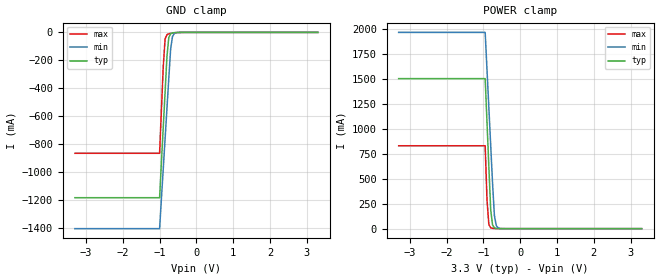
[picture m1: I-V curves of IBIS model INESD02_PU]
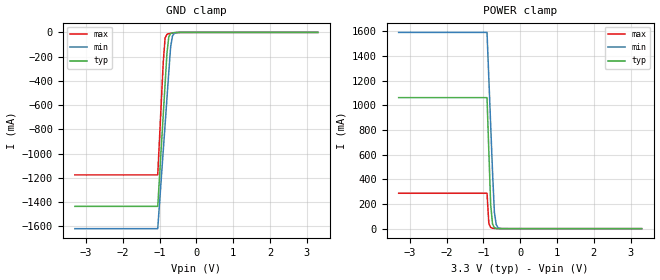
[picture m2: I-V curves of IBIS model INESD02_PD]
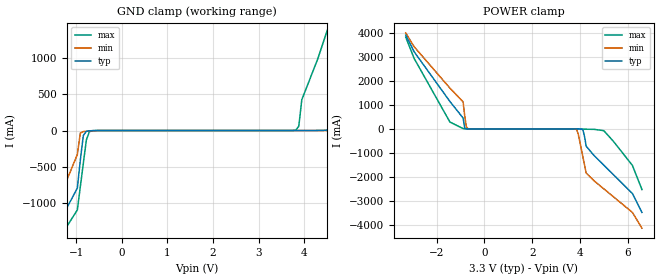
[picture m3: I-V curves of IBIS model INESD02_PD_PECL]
|   This file is an IBIS representation of the   |
|   Integrated Device Technology, Inc.   |
|   ICS85105I   |
|   Low Skew, 1-to-5, Differential/LVCMOS-to-0.7V HCSL Fanout Buffer   |
[IBIS Ver]   4.1
[File name]   85105i_3v3.ibs
[File Rev]   4.0
[Date]   27 Aug 2009 | Last modified
|   May 07 2007 | Generated
[Source]   Originated at Integrated Device Technology, Inc.
[Disclaimer]
IDT hereby grants the user of this IBIS model a non-exclusive,
nontransferable license to use this IBIS model under the following terms.
Before using this IBIS model, the user should read this license.
If the user does not accept these terms,  the IBIS model should be
returned to IDT within 30 days.
   The user is granted this license only to use the IBIS model and
is not granted rights to sell, load, rent, lease or license the IBIS
model in whole or in part, or in modified form to anyone other than
user. User may modify the IBIS model to suit its specific
applications but rights to derivative works and such modifications
shall belong to IDT.
   This IBIS model is provided on an "AS IS" basis and IDT makes
absolutely no warranty with respect to the information contained
herein. IDT DISCLAIMS AND CUSTOMER WAIVES ALL WARRANTIES, EXPRESS
OR IMPLIED, INCLUDING WARRANTIES OF MERCHANTABILITY OR FITNESS FOR
A PARTICULAR PURPOSE. The entire risk as to quality and performance
is with the Customer. ACCORDINGLY, IN NO EVENT SHALL THE COMPANY BE
LIABLE FOR ANY DAMAGES, WHETHER IN CONTRACT OR TORT,INCLUDING ANY
LOST PROFITS OR OTHER INCIDENTAL, CONSEQUENTIAL, EXEMPLARY, OR
PUNITIVE DAMAGES ARISING OUT OF THE USE OR APPLICATION OF THE IBIS
model provided in this package. Further, IDT reserves the right to
make changes without notice to any product herein to improve
reliability, function, or design. IDT does not convey any license
under patent rights or any other intellectual property rights,
including those of third parties.
   IDT is not obligated to provide maintenance or support
for the licensed IBIS model.
[Copyright]   Copyright 2006 by Integrated Device Technology, Inc.
[Component]   ICS85105GI
[Manufacturer] Integrated Device Technology, Inc.
[Package]
|TSSOP 20 Lead
|   typ   min   max
R_pkg   51.85m   41.1m   62.6m
L_pkg   1.568nH   0.734nH   2.401nH
C_pkg   0.221pF   0.068pF   0.373pF
[Pin] signal_name  model_name   R_pin   L_pin   C_pin
1   GND   GND   62.6m   2.401n   0.373p
2   CLK_EN   INESD02_PU   57.23m   1.985n   0.297p
3   CLK_SEL   INESD02_PD   51.85m   1.568n   0.221p
4   CLK0   INESD02_PD_PECL   46.78m   1.151n   0.145p
5   nCLK0   INESD02_PD_PU   41.1m   0.734n   0.068p
6   CLK1   INESD02_PD_PECL   41.1m   0.734n   0.068p
7   Q4   DCMOUT01_ISO2_OP   46.78m   1.151n   0.145p
8   nQ4   DCMOUT01_ISO2_OP   51.85m   1.568n   0.221p
9   IREF   NC   57.23m   1.985n   0.297p
10  VDD   POWER   62.6m   2.401n   0.373p
11  nQ3   DCMOUT01_ISO2_OP   62.6m   2.401n   0.373p
12  Q3   DCMOUT01_ISO2_OP   57.23m   1.985n   0.297p
13  VDD   POWER   51.85m   1.568n   0.221p
14  nQ2   DCMOUT01_ISO2_OP   46.78m   1.151n   0.145p
15  Q2   DCMOUT01_ISO2_OP   41.1m   0.734n   0.068p
16  nQ1   DCMOUT01_ISO2_OP   41.1m   0.734n   0.068p
17  Q1   DCMOUT01_ISO2_OP   46.78m   1.151n   0.145p
18  VDD   POWER   51.85m   1.568n   0.221p
19  nQ0   DCMOUT01_ISO2_OP   57.23m   1.985n   0.297p
20  Q0   DCMOUT01_ISO2_OP   62.6m   2.401n   0.373p
[Diff Pin]   inv_pin  vdiff tdelay_typ tdelay_min  tdelay_max
   4   5   0.15   0   0   0
   20   19   NA   0   0   0
   17   16   NA   0   0   0
   15   14   NA   0   0   0
   12   11   NA   0   0   0
   7   8   NA   0   0   0
| Models and submodels in the file (5): INESD02_PU (Input), INESD02_PD (Input), INESD02_PD_PECL (Input), INESD02_PD_PU (Input), DCMOUT01_ISO2_OP (Open_source)
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[Model]   INESD02_PU
Model_type   Input
Polarity   Non-Inverting
Vinl = 0.80V
Vinh = 2.0V
|   typ   min   max
C_comp   2pF   1.5pF   2.5pF
|   typ   min   max
[Voltage range]  3.3V   3.15V   3.45V
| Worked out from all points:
|   GND clamp passes 1 mA (typ) near -0.56 V on its own axis
|   POWER clamp passes 1 mA (typ) near -0.61 V on its own axis
[GND_clamp]
|Voltage   I(typ)   I(min)   I(max)
-3.3V     -1.184A    -1.405A    -865.6mA
-1V       -1.184A    -1.405A    -865.6mA
-900mV    -678.5mA   -975.1mA   -244.1mA
-850mV    -426.2mA   -760.2mA   -46.92mA
-800mV    -174mA     -545.4mA   -16.17mA
-750mV    -37.03mA   -330.8mA   -9.981mA
-700mV    -9.767mA   -120.3mA   -7.122mA
-650mV    -3.616mA   -29.78mA   -4.922mA
-600mV    -1.7mA     -7.594mA   -3.115mA
-400mV    -123.9uA   -126uA     -173.9uA
3.3V      1.866nA    3.949uA    0A
[POWER_clamp]
|Voltage   I(typ)   I(min)   I(max)
-3.3V     1.506A     1.97A      832.1mA
-950mV    1.506A     1.97A      832.1mA
-900mV    1.063A     1.592A     287.2mA
-850mV    620.4mA    1.215A     41.77mA
-800mV    191.5mA    837.4mA    8.692mA
-750mV    37.69mA    460.1mA    3.262mA
-700mV    8.032mA    133.8mA    1.662mA
-650mV    2.005mA    32.58mA    840.1uA
-600mV    607uA      8.009mA    378.6uA
-450mV    33.11uA    139.8uA    23.88uA
3.3V      -71.13uA   -77.46uA   -62.11uA
[Model]   INESD02_PD
Model_type   Input
Polarity   Non-Inverting
Vinl = 0.80V
Vinh = 2.0V
|   typ   min   max
C_comp   2pF   1.5pF   2.5pF
|   typ   min   max
[Voltage range]  3.3V   3.15V   3.45V
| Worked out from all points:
|   GND clamp passes 1 mA (typ) near -0.56 V on its own axis
|   POWER clamp passes 1 mA (typ) near -0.61 V on its own axis
[GND_clamp]
|Voltage   I(typ)   I(min)   I(max)
-3.3V     -1.436A    -1.62A     -1.176A
-1.05V    -1.436A    -1.62A     -1.176A
-900mV    -678.5mA   -975.1mA   -244mA
-850mV    -426.1mA   -760.1mA   -46.85mA
-800mV    -173.9mA   -545.4mA   -16.11mA
-750mV    -36.96mA   -330.7mA   -9.916mA
-700mV    -9.696mA   -120.2mA   -7.056mA
-650mV    -3.545mA   -29.7mA    -4.857mA
-600mV    -1.629mA   -7.52mA    -3.049mA
-400mV    -52.81uA   -52.52uA   -108.7uA
3.3V      71.13uA    77.43uA    62.11uA
[POWER_clamp]
|Voltage   I(typ)   I(min)   I(max)
-3.3V     1.063A     1.593A     287.3mA
-900mV    1.063A     1.593A     287.3mA
-850mV    620.5mA    1.215A     41.84mA
-800mV    191.6mA    837.5mA    8.757mA
-750mV    37.76mA    460.2mA    3.328mA
-700mV    8.104mA    133.8mA    1.728mA
-650mV    2.076mA    32.66mA    905.3uA
-600mV    678.1uA    8.083mA    443.8uA
-450mV    104.2uA    213.3uA    89.09uA
3.3V      -3.041nA   -3.986uA   0A
[Model]   INESD02_PD_PECL
Model_type  Input
Polarity   Non-Inverting
Vinl = 0.8V
Vinh = 2.0V
|   typ   min   max
C_comp   2pF   1.5pF   2.5pF
|   typ   min   max
[Voltage range]  3.3V   3.15V   3.45V
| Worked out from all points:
|   GND clamp passes 1 mA (typ) near -0.59 V on its own axis
|   POWER clamp passes 1 mA (typ) near -0.70 V on its own axis
[GND_clamp]
-3.3V     -3.894A    -4.294A    -3.674A
-1.6V     -1.569A    -1.322A    -1.74A
-974.8mV  -794.1mA   -331.5mA   -1.096A
-843.4mV  -68.33mA   -15.34mA   -452.9mA
-646.5mV  -1.912mA   -4.151mA   -2.665mA
3.818V    89.38uA    70.49uA    7.198mA
3.95V     342.2uA    75.94uA    423.8mA
4.6V      7.437mA    165.5uA    1.553A
4.9V      78.32mA    440.9uA    2.118A
5.5V      1.293A     2.769mA    3.249A
6.25V     2.651A     112.4mA    4.38A
6.6V      3.331A     896.1mA    4.946A
[POWER_clamp]
-3.3V     3.923A     4.017A     3.838A
-2.95V    3.23A      3.44A      2.951A
-1.45V    1.149A     1.709A     289.6mA
-896.9mV  456.5mA    1.133A     15.4mA
-762.9mV  4.223mA    91.07mA    1.486mA
-695.9mV  792.2uA    10.73mA    555.6uA
3.861V    -556.7uA   -26.14mA   -39.45uA
4.129V    -41.85mA   -1.19A     -4.904mA
4.263V    -724.2mA   -1.847A    -12.04mA
5V        -1.514A    -2.505A    -71.38mA
6.2V      -2.701A    -3.492A    -1.525A
6.6V      -3.492A    -4.151A    -2.536A
